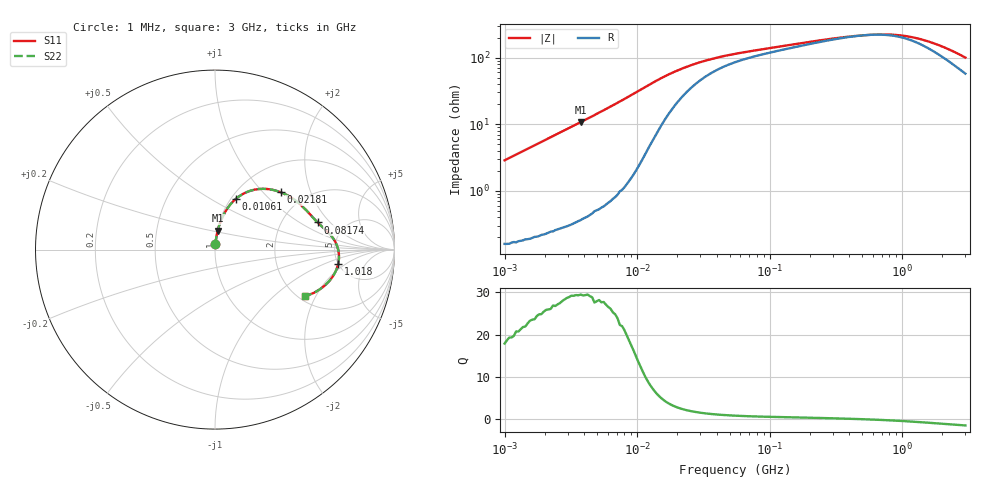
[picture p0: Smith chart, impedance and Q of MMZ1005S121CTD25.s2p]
! S-Parameter Data Generated by TDK Corporation
! Copyright(C) 2025 TDK Corporation.
! All Rights Reserved.
! TDK P/N: MMZ1005S121CTD25 (Chip Bead)
! Property: |Z|=120ohm at 100MHz
! Size(LxWxT): 1x0.5x0.5mm
! Model Type: s2p (Touchstone File Format Version 1.0)
! Frequency: DC=Yes Start=1MHz Stop=3000MHz 202points Log-sweep
! Model Generated on Feb. 6, 2025
! Terms and conditions regarding TDK Simulation Models:
! 1)This simulation model is being provided solely for informational
!  purposes. Please refer to the specifications of the products in
!  terms of detailed characteristics of such products.
! 2)In no event shall TDK Corporation of any of its subsidiaries be
!  liable for any loss or damage arising, directly or indirectly,
!  from any information contained in this simulation model, including,
!  but not limited to loss or damages arising from any inaccuracies,
!  omissions or errors in connection with such information.
! 3)Any and all copyrights on this simulation model are owned by
!  TDK Corporation.  Duplication or redistribution of this simulation
!  model without prior written permission from TDK Corporation
!  is prohibited.
! 4)This simulation model is subject to any modification or change
!  without any prior notice.
! 5)Neither TDK Corporation nor any of its subsidiaries shall make any
!  warranty, express or implied, including but not limited to the
!  correctness, implied warranties of merchantability and fitness for
!  a particular purpose with respect to this simulation models.
! 6)The use of this simulation model shall be deemed to have consented
!  to the terms and conditions hereof.
! Port Assignments:
!  1 ---@@@--- 2
! Applicable Conditions:
!  Temperature = 25 degC
!  DC Bias Current = 0 A
!  Small Signal Operation
# Hz S MA R 50
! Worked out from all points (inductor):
!   201 points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, 1 MHz to 3 GHz, reference 50 ohm
!   read as one part in series: L = 457 nH near 1.041 MHz
!   highest Q = 29.3 at 3.747 MHz (marker M1), where L = 457 nH
!   self-resonance near 557.2 MHz
!   S11 on the Smith chart (normalised r, x): 1 MHz: 1.00, +0.06; 10.61 MHz: 1.05, +0.66; 21.81 MHz: 1.51, +1.27; 81.74 MHz: 3.15, +1.47; 1.018 GHz: 4.97, -1.54; 3 GHz: 2.15, -1.64
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1000000  0.02873 85.2  0.998 -1.6  0.998 -1.6  0.02873 85.2
2055611  0.05871 84.4  0.996 -3.4  0.996 -3.4  0.05871 84.4
3747356  0.1066 81.9  0.9907 -6.1  0.9907 -6.1  0.1066 81.9
3900413  0.111 81.7  0.99 -6.4  0.99 -6.4  0.111 81.7
7110411  0.2034 75.9  0.9706 -11.7  0.9706 -11.7  0.2034 75.9
8686058  0.2498 72.5  0.955 -14.4  0.955 -14.4  0.2498 72.5
1.061086e7  0.3056 67.7  0.928 -17.7  0.928 -17.7  0.3056 67.7
1.461624e7  0.4002 56.6  0.8479 -23.2  0.8479 -23.2  0.4002 56.6
1.785516e7  0.4489 48.6  0.7799 -25.6  0.7799 -25.6  0.4489 48.6
2.181181e7  0.4856 41.2  0.7106 -26.7  0.7106 -26.7  0.4856 41.2
2.664524e7  0.5129 34.7  0.6475 -26.8  0.6475 -26.8  0.5129 34.7
3.387922e7  0.5365 28.2  0.585 -25.7  0.585 -25.7  0.5365 28.2
5.477226e7  0.569 19.4  0.5003 -22.2  0.5003 -22.2  0.569 19.4
8.173662e7  0.5915 14.8  0.4541 -19.5  0.4541 -19.5  0.5915 14.8
2.136344e8  0.6468 7.5  0.3686 -13.3  0.3686 -13.3  0.6468 7.5
4.75755e8  0.6816 1.4  0.319 -3.1  0.319 -3.1  0.6816 1.4
8.005644e8  0.6921 -3.7  0.3126 8.3  0.3126 8.3  0.6921 -3.7
1.017911e9  0.6906 -6.7  0.3245 14.5  0.3245 14.5  0.6906 -6.7
1.347129e9  0.6806 -10.9  0.356 21.3  0.356 21.3  0.6806 -10.9
1.782824e9  0.6573 -15.9  0.4095 26.1  0.4095 26.1  0.6573 -15.9
2.266846e9  0.6239 -20.8  0.4723 28.0  0.4723 28.0  0.6239 -20.8
3e9  0.5636 -27.5  0.5635 27.5  0.5635 27.5  0.5636 -27.5
